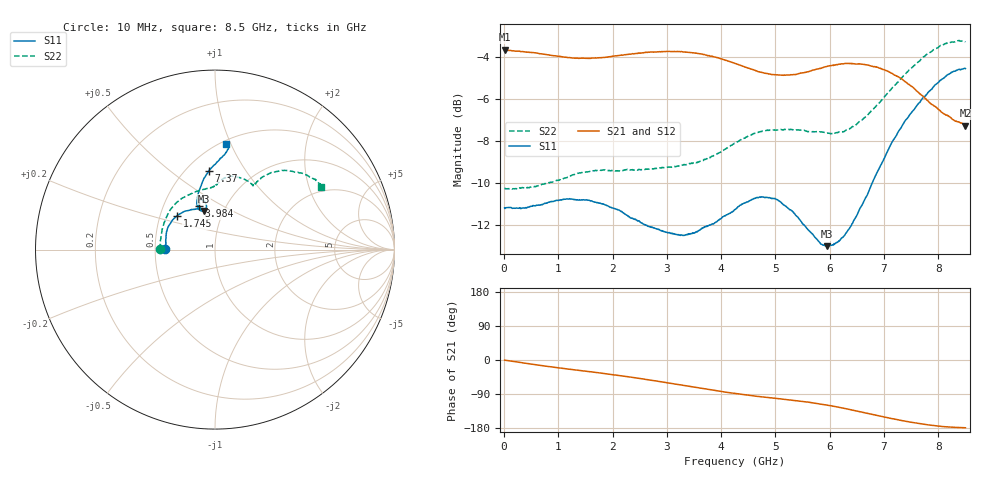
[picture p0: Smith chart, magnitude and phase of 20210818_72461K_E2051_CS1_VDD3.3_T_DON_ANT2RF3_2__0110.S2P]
!Agilent Technologies,E5071C,MY46417908,A.11.23
!Date: Wed Aug 18 14:30:00 2021
!Data & Calibration Information:
!Freq	S11:SOLT2(ON)	S21:SOLT2(ON)	S12:SOLT2(ON)	S22:SOLT2(ON)
!PortZ  Port1:50+j0  Port2:50+j0
!Above PortZ is port z conversion or system Z0 setting when saving the data.
!When reading, reference impedance value at option line is always used.
# Hz S dB R 50
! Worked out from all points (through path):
!   1601 points, 10 MHz to 8.5 GHz, reference 50 ohm
!   highest |S21| = -3.65 dB at 10 MHz (marker M1); lowest = -7.3 dB at 8.5 GHz (marker M2)
!   group delay of S21, straight-line fit = 59.9 ps
!   lowest |S11| = -13.0 dB at 5.953 GHz (marker M3), VSWR 1.58, Z = 40.6 + j18.4 ohm
!   |S11| at or under -10 dB: start of sweep to 6.782 GHz
!   |S22| runs from -10.3 to -3.2 dB; largest |S21 - S12| = 0.0036
!   S11 on the Smith chart (normalised r, x): 10 MHz: 0.57, +0.00; 1.745 GHz: 0.61, +0.25; 3.984 GHz: 0.75, +0.39; 7.37 GHz: 0.64, +0.70; 8.5 GHz: 0.53, +0.96
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1e7  -11.19 179.6  -3.65 -0.4  -3.65 -0.4  -10.24 179.8
7.900188e8  -10.96 164.0  -3.88 -16.6  -3.88 -16.6  -10.01 157.5
1.426769e9  -10.80 147.8  -4.05 -28.2  -4.05 -28.2  -9.50 136.4
1.745144e9  -10.96 138.7  -4.03 -33.8  -4.03 -33.8  -9.38 125.7
2.328831e9  -11.66 123.1  -3.86 -45.1  -3.86 -45.1  -9.38 108.4
2.843538e9  -12.21 112.6  -3.74 -56.4  -3.74 -56.4  -9.29 97.2
3.411306e9  -12.41 109.2  -3.77 -69.5  -3.76 -69.6  -9.07 91.2
3.984381e9  -11.71 110.4  -4.07 -82.7  -4.06 -82.8  -8.53 86.7
4.255e9  -11.26 110.0  -4.29 -88.4  -4.29 -88.5  -8.10 84.0
4.63705e9  -10.71 108.4  -4.65 -95.5  -4.64 -95.5  -7.62 78.8
4.997875e9  -10.75 104.9  -4.84 -101.0  -4.84 -101.0  -7.47 72.0
5.671769e9  -12.40 101.7  -4.64 -112.5  -4.65 -112.6  -7.56 61.3
5.953e9  -13.01 105.7  -4.44 -118.9  -4.45 -119.0  -7.62 59.8
6.218312e9  -12.62 110.8  -4.32 -126.1  -4.32 -126.3  -7.56 59.3
6.473012e9  -11.66 112.0  -4.32 -133.9  -4.31 -134.0  -7.23 58.4
6.733019e9  -10.30 108.6  -4.40 -142.1  -4.38 -142.2  -6.65 57.3
7.088538e9  -8.35 100.7  -4.69 -153.0  -4.70 -153.0  -5.65 54.4
7.369769e9  -7.11 94.3  -5.12 -160.9  -5.11 -161.0  -4.86 50.3
7.709369e9  -5.96 87.1  -5.83 -169.1  -5.83 -169.2  -4.02 43.2
8.017131e9  -5.15 83.1  -6.51 -174.9  -6.47 -174.9  -3.49 37.0
8.346119e9  -4.62 83.0  -7.07 -178.0  -7.04 -177.9  -3.22 32.0
8.5e9  -4.54 84.0  -7.27 -178.8  -7.21 -178.7  -3.28 30.7
